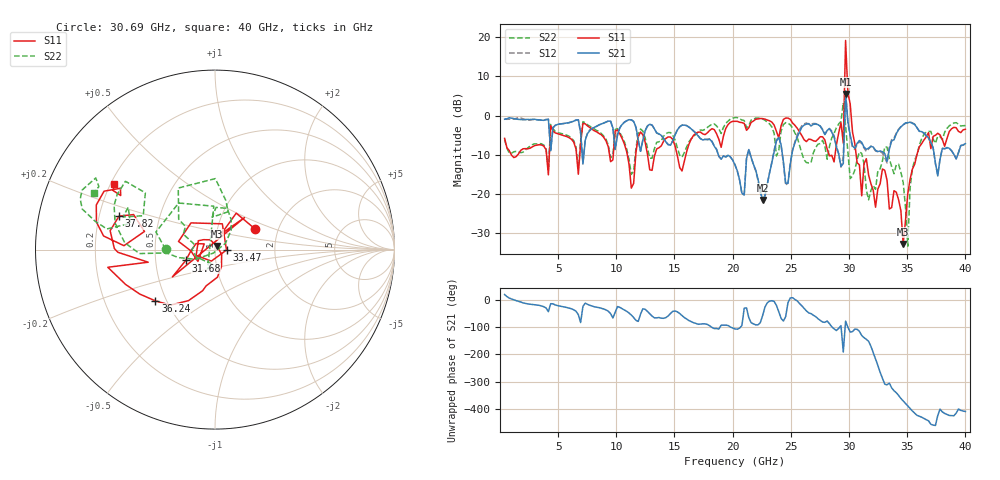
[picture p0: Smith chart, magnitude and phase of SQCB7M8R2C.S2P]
! Network Analyzer HP8722ES.07.66: Jul 25, 2000 Serial No. US39175408
! 26 Oct 2004  15:45:27
! Frequency  S11  S21  S12  S22
# HZ  S  DB R  50
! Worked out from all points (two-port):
!   201 points, 400 MHz to 40 GHz, reference 50 ohm
!   highest |S21| = 5.52 dB at 29.7 GHz (marker M1); lowest = -21.5 dB at 22.58 GHz (marker M2)
!   |S21| within 3 dB of the highest: 29.67057 GHz to 29.78746 GHz (116.9 MHz wide, 0.393 % of centre)
!   lowest |S11| = -32.7 dB at 34.65 GHz (marker M3), VSWR 1.05, Z = 51 + j2.11 ohm
!   |S11| at or under -10 dB: 974.6 MHz to 1.532 GHz (557.8 MHz wide, 44.5 % of centre); 15.23 GHz to 15.98 GHz (754.3 MHz wide, 4.83 % of centre); 30.61 GHz to 35.83 GHz (5.22 GHz wide, 15.7 % of centre)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
!   |S22| runs from -33.3 to 3.2 dB; largest |S21 - S12| = 0.71
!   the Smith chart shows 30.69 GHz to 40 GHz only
!   S11 on the Smith chart (normalised r, x): 30.69 GHz: 1.51, +0.38; 31.68 GHz: 0.72, -0.09; 33.47 GHz: 1.14, -0.01; 36.24 GHz: 0.44, -0.31; 37.82 GHz: 0.28, +0.16; 40 GHz: 0.22, +0.28
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4e8  -5.84 -71.5  -0.94 21.2  -0.87 24.6  -6.15 -64.8
4.162e9  -15.12 -114.6  -0.97 -42.1  -0.94 -42.2  -14.20 -112.2
4.36e9  -2.59 -71.9  -8.99 -12.6  -8.86 -9.5  -2.27 -73.4
7.132e9  -1.97 -77.5  -12.38 -22.2  -12.17 -21.0  -1.56 -76.5
1.129e10  -18.51 -112.9  -1.09 -54.5  -1.08 -54.7  -15.02 -93.9
1.3666e10  -8.21 -46.5  -4.68 -63.6  -4.74 -63.4  -6.69 -42.0
2.02e10  -1.49 -18.4  -12.59 -105.7  -12.52 -105.3  -0.52 -12.7
2.2576e10  -0.79 -27.5  -21.53 -56.1  -22.06 -55.3  -0.90 -28.2
2.515e10  -1.91 -47.5  -8.81 9.5  -8.85 7.9  -3.20 -65.5
2.6932e10  -6.44 -50.5  -2.26 -55.1  -2.04 -54.9  -9.54 113.4
2.8714e10  -11.82 -32.3  -5.51 -105.5  -5.13 -106.2  -4.55 72.3
2.9506e10  -7.04 7.9  -12.25 169.0  -10.55 -153.3  3.24 24.0
2.9704e10  19.14 -33.5  5.52 -77.0  6.30 -57.0  -2.57 -77.5
2.9902e10  5.72 -120.9  -1.59 -99.7  -1.88 -102.4  -9.37 -26.1
3.0694e10  -12.04 27.9  -7.10 -107.3  -7.42 -107.4  -11.22 179.8
3.1684e10  -15.21 -159.7  -8.34 -151.7  -8.50 -149.5  -21.48 -97.2
3.3466e10  -23.83 -2.1  -8.57 54.1  -8.04 55.6  -11.07 77.4
3.4654e10  -32.73 63.8  -2.40 -11.5  -2.35 -11.0  -17.03 50.1
3.505e10  -19.88 -69.2  -1.84 -30.0  -1.80 -30.4  -33.31 -115.7
3.6238e10  -7.17 -139.4  -4.10 -71.5  -4.17 -70.8  -5.94 175.7
3.7822e10  -4.94 160.7  -11.13 -41.7  -11.00 -41.9  -5.38 154.0
4e10  -3.50 147.0  -7.17 -50.6  -7.19 -49.3  -2.55 154.9
